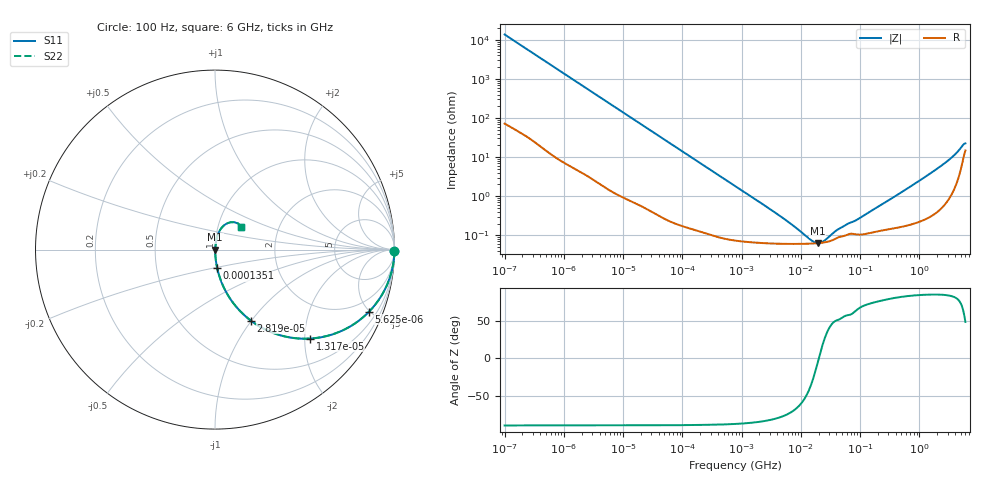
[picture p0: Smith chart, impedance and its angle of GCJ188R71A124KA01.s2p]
!Murata Part Number: GCJ188R71A124KA01
!These Parameters are Measured in Series Mode Connection
!Data Generated on Mar 13, 2026
!  o--ll--o
!Port1  Port2
!  o------o
!Operation Temp=25[degC], DC Bias Voltage=0[V]
!Freq. Start=100[Hz] Stop=6[GHz] 401[Steps]
# Hz S RI R 50
!Freq.(Hz) S11(Real) S11(Imag) S21(Real) S21(Imag) S12(Real) S12(Imag) S22(Real) S22(Imag)
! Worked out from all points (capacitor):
!   401 points, 100 Hz to 6 GHz, reference 50 ohm
!   read as one part in series: C = 116 nF near 109 Hz
!   lowest |Z| = 63.3 mohm at 19.46 MHz (marker M1)
!   series resonance near 20.09 MHz, so ESL is about 540 pH
!   S11 on the Smith chart (normalised r, x): 100 Hz: open; 5.625 kHz: 1.03, -4.95; 13.17 kHz: 1.02, -2.12; 28.19 kHz: 1.01, -0.99; 135.1 kHz: 1.00, -0.21; 6 GHz: 1.30, +0.34
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100  0.9999 -0.00728  9.14e-05 0.00728  9.14e-05 0.00728  0.9999 -0.00728
600  0.9979 -0.0433  0.0021 0.0433  0.0021 0.0433  0.9979 -0.0433
2008  0.9787 -0.1416  0.0213 0.1416  0.0213 0.1416  0.9787 -0.1416
5625  0.8582 -0.3459  0.1418 0.3459  0.1418 0.3459  0.8582 -0.3459
8416  0.7315 -0.44  0.2685 0.44  0.2685 0.44  0.7315 -0.44
13169  0.5289 -0.4956  0.4711 0.4956  0.4711 0.4956  0.5289 -0.4956
18841  0.3563 -0.4749  0.6437 0.4749  0.6437 0.4749  0.3563 -0.4749
28191  0.2002 -0.3959  0.7998 0.3959  0.7998 0.3959  0.2002 -0.3959
40335  0.1102 -0.3087  0.8898 0.3087  0.8898 0.3087  0.1102 -0.3087
135116  0.0122 -0.103  0.9878 0.103  0.9878 0.103  0.0122 -0.103
774597  0.00107 -0.0184  0.9989 0.0184  0.9989 0.0184  0.00107 -0.0184
5079039  0.000613 -0.00265  0.9994 0.00265  0.9994 0.00265  0.000613 -0.00265
1.555665e7  0.000617 -0.000372  0.9994 0.000372  0.9994 0.000372  0.000617 -0.000372
1.946e7  0.000631 -4.58e-05  0.9994 4.58e-05  0.9994 4.58e-05  0.000631 -4.58e-05
2.434276e7  0.000656 0.000279  0.9993 -0.000279  0.9993 -0.000279  0.000656 0.000279
4.165952e7  0.000873 0.00109  0.9991 -0.00109  0.9991 -0.00109  0.000873 0.00109
8.918374e7  0.00105 0.00228  0.9989 -0.00228  0.9989 -0.00228  0.00105 0.00228
3.124326e8  0.0015 0.00794  0.9985 -0.00794  0.9985 -0.00794  0.0015 0.00794
1.431855e9  0.00407 0.0354  0.9959 -0.0354  0.9959 -0.0354  0.00407 0.0354
3.352442e9  0.0177 0.0888  0.9823 -0.0888  0.9823 -0.0888  0.0177 0.0888
4.586474e9  0.0472 0.1323  0.9528 -0.1323  0.9528 -0.1323  0.0472 0.1323
6e9  0.1473 0.126  0.8527 -0.126  0.8527 -0.126  0.1473 0.126
